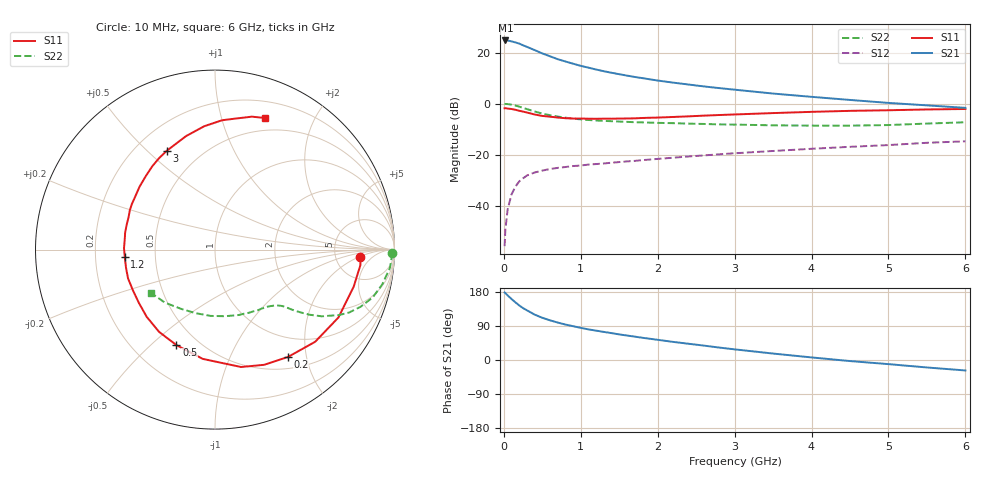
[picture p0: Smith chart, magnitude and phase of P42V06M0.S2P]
! SIEMENS Small Signal Semiconductors
! BFP182
! Si NPN RF Bipolar Junction Transistor in SOT143
! VCE = 2 V  IC = 6 mA
! Common Emitter S-Parameters:  March  1996
# GHz  S  MA  R  50
!  f  S11  S21  S12  S22
! GHz  MAG  ANG  MAG  ANG  MAG  ANG  MAG  ANG
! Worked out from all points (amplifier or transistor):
!   36 points, 10 MHz to 6 GHz, reference 50 ohm
!   highest |S21| = 24.8 dB at 20 MHz (marker M1)
!   |S21| within 3 dB of that: start of sweep to 338.6 MHz
!   unconditionally stable (mu >= 1): 1.437 GHz to 5.482 GHz
!   at 250 MHz: K = 0.24, MSG = 26.1 dB, |S12| = -29.3 dB
!   at 1.4 GHz: K = 0.99, MSG = 17.6 dB, |S12| = -23.2 dB
!   at 6 GHz: K = 0.96, MSG = 6.6 dB, |S12| = -14.8 dB
!   lowest NFmin = 1.25 dB at 450 MHz
!   S11 on the Smith chart (normalised r, x): 10 MHz: 9.07, -2.18; 200 MHz: 0.67, -1.69; 500 MHz: 0.38, -0.60; 1.2 GHz: 0.33, -0.04; 3 GHz: 0.33, +0.58; 6 GHz: 0.36, +1.39
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0.01  0.8113 -2.9  17.28 178.2  0.0016 85.4  0.9888 -1.1
0.02  0.8147 -6.1  17.34 176.6  0.0034 80.9  0.9861 -2.3
0.05  0.7998 -15.0  17.3 170.3  0.0085 84.2  0.9798 -6.0
0.1  0.7848 -28.8  16.63 160.9  0.0166 73.8  0.9516 -11.8
0.15  0.7585 -42.6  15.87 152.2  0.0235 68.2  0.9181 -16.9
0.2  0.7233 -55.8  15.05 144.0  0.0298 63.2  0.8719 -21.4
0.25  0.6978 -66.9  13.93 136.9  0.0343 58.1  0.8259 -25.1
0.3  0.67 -77.5  12.99 131.1  0.0389 54.4  0.7816 -27.8
0.4  0.6127 -96.4  11.23 119.8  0.0446 47.8  0.7014 -32.0
0.5  0.5738 -112.0  9.653 111.4  0.0486 43.0  0.6388 -34.6
0.6  0.5542 -124.2  8.486 104.7  0.0522 40.7  0.593 -36.2
0.7  0.534 -135.4  7.45 98.8  0.0549 39.2  0.5579 -37.5
0.9  0.5104 -153.8  6.073 89.2  0.0597 36.8  0.5074 -39.1
1.1  0.506 -168.6  5.074 80.8  0.0638 36.2  0.478 -40.8
1.2  0.5043 -175.2  4.663 77.5  0.0653 35.8  0.4672 -41.8
1.7  0.5144 159.3  3.337 61.7  0.0753 36.1  0.4324 -47.3
2.2  0.5475 140.1  2.583 47.8  0.0869 35.5  0.4139 -54.7
3  0.613 115.9  1.878 28.1  0.1063 33.0  0.3877 -70.0
3.5  0.6527 104.3  1.576 17.0  0.1178 30.4  0.3754 -81.3
4.5  0.7216 86.9  1.181 -2.8  0.1422 25.1  0.3702 -107.0
5.5  0.7686 74.5  0.925 -19.7  0.1706 18.8  0.4065 -133.4
6  0.7849 69.1  0.826 -27.6  0.1824 14.5  0.4307 -146.0
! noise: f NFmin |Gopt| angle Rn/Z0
0.45  1.25  0.25  39  0.3
0.9  1.4  0.25  78  0.23
1.8  1.95  0.21  151  0.2
